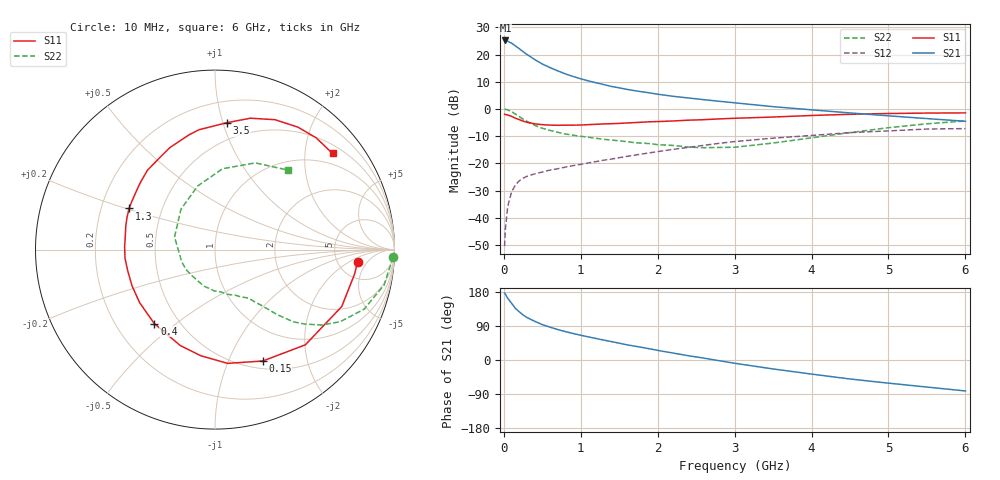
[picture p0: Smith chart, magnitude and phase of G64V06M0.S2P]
! SIEMENS Small Signal Semiconductors
! BFG193
! Si NPN RF Bipolar Junction Transistor in SOT223
! VCE = 4 V  IC = 6 mA
! Common Emitter S-Parameters:  August  1996
# GHz  S  MA  R  50
!  f  S11  S21  S12  S22
! GHz  MAG  ANG  MAG  ANG  MAG  ANG  MAG  ANG
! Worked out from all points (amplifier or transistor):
!   36 points, 10 MHz to 6 GHz, reference 50 ohm
!   highest |S21| = 25.2 dB at 20 MHz (marker M1)
!   |S21| within 3 dB of that: start of sweep to 199.3 MHz
!   unconditionally stable (mu >= 1): 1.035 GHz to 2.553 GHz
!   at 250 MHz: K = 0.38, MSG = 23.3 dB, |S12| = -25.5 dB
!   at 1.4 GHz: K = 1.08, MAG = 11.6 dB, |S12| = -18.4 dB
!   at 6 GHz: K = 0.87, MSG = 1.4 dB, |S12| = -7.2 dB
!   S11 on the Smith chart (normalised r, x): 10 MHz: 7.77, -2.91; 150 MHz: 0.59, -1.34; 400 MHz: 0.37, -0.42; 1.3 GHz: 0.32, +0.20; 3.5 GHz: 0.36, +1.03; 6 GHz: 0.70, +2.64
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0.01  0.7976 -4.9  18.09 176.4  0.003 88.9  0.9908 -2.4
0.02  0.7894 -10.0  18.16 173.9  0.0062 86.1  0.9823 -4.8
0.05  0.7742 -24.2  17.63 162.9  0.016 78.0  0.9627 -11.8
0.1  0.7313 -46.5  16.21 149.9  0.0297 68.8  0.8943 -21.8
0.15  0.6753 -66.8  14.43 136.3  0.04 59.2  0.8043 -30.0
0.2  0.6377 -83.7  12.83 127.3  0.0477 54.0  0.7258 -35.4
0.25  0.5967 -97.6  11.33 118.8  0.0532 49.7  0.6493 -39.7
0.3  0.5684 -109.9  10.06 112.2  0.0577 47.2  0.5928 -42.7
0.4  0.5332 -129.3  8.121 102.2  0.064 43.7  0.5007 -46.3
0.5  0.5136 -144.8  6.697 93.4  0.0693 42.0  0.4418 -48.5
0.6  0.5045 -156.4  5.757 86.7  0.0752 41.6  0.4029 -50.3
0.7  0.5003 -166.4  5.014 80.4  0.0795 41.7  0.3722 -52.4
0.9  0.5038 178.0  3.957 69.9  0.0908 42.2  0.3284 -55.5
1.1  0.5145 165.1  3.275 61.0  0.1017 42.3  0.3016 -61.2
1.3  0.5308 154.4  2.803 52.5  0.1144 42.1  0.2765 -66.3
1.6  0.5526 140.6  2.29 40.1  0.1343 40.4  0.2503 -77.6
2.2  0.6008 119.9  1.708 18.3  0.1805 33.8  0.2134 -106.3
2.8  0.6565 102.5  1.383 -1.9  0.2331 24.1  0.196 -145.6
3.5  0.71 84.7  1.101 -23.6  0.2904 9.0  0.2362 162.7
4.5  0.7973 65.2  0.845 -50.1  0.3675 -11.4  0.367 105.3
5.5  0.8398 47.9  0.665 -71.4  0.4272 -36.9  0.5331 65.0
6  0.846 39.3  0.593 -81.7  0.4344 -51.5  0.601 47.5
